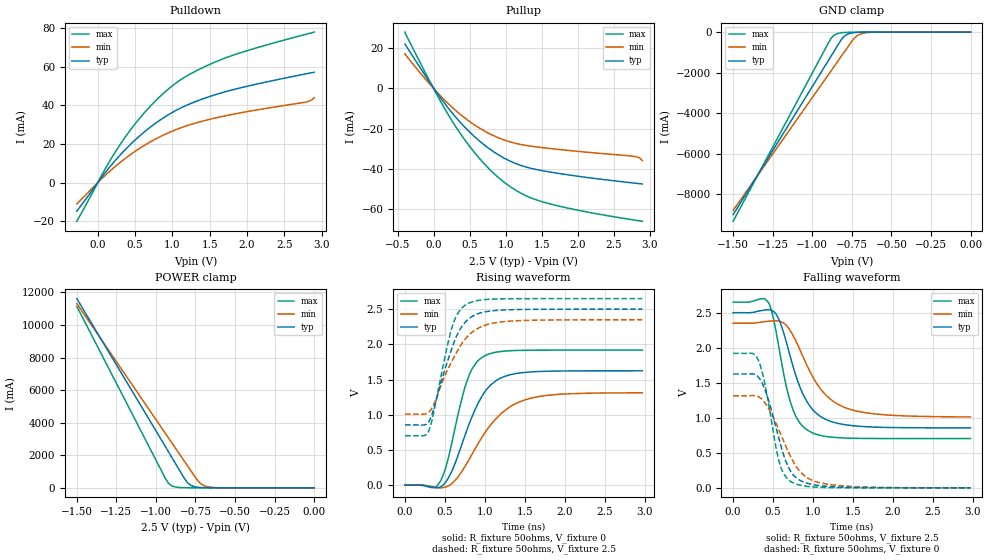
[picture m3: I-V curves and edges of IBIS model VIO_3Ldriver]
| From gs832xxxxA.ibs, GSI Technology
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|  signals   DQA1-DQA9, DQB1-DQB9, DQC1-DQC9, DQD1-DQD9
[Model]   VIO_3Ldriver
Model_type   I/O
Polarity   Non-Inverting
Vinl  =   0.80v
Vinh  =   2.00v
Vmeas =   1.25v
Cref  =   0pF
Rref  =   50
Vref  =   1.25v
|  variable   typ   min   max
C_comp   3.0pF   2.5pF   3.5pF
|  variable   typ   min   max
[Temperature Range]   50   0   100
|  variable   typ   min   max
[Voltage Range]   2.5   2.35   2.65
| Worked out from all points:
|   slope of the pulldown table from 0 to 0.375 V, typ, clamps not added: 21.6 ohm
|   slope of the pullup table from 0 to 0.375 V, typ, clamps not added: 21.9 ohm
|   GND clamp passes 1 mA (typ) near -0.58 V on its own axis
|   POWER clamp passes 1 mA (typ) near -0.61 V on its own axis
|   rising waveform, R_fixture 50ohms, V_fixture 0: 20-80 % time 352ps typ, 488ps min, 252ps max; typ from 0 V to 1.62 V
|   rising waveform, R_fixture 50ohms, V_fixture 2.5: 20-80 % time 284ps typ, 353ps min, 224ps max; typ from 0.855 V to 2.5 V
|   falling waveform, R_fixture 50ohms, V_fixture 2.5: 20-80 % time 308ps typ, 411ps min, 225ps max; typ from 2.5 V to 0.856 V
|   falling waveform, R_fixture 50ohms, V_fixture 0: 20-80 % time 250ps typ, 334ps min, 186ps max; typ from 1.62 V to 0 V
[Pulldown]
| voltage   typ   min   max
-280mV    -14.72mA   -10.94mA   -19.96mA
105mV     5.397mA    3.94mA     7.47mA
350mV     16.36mA    11.99mA    22.57mA
525mV     22.94mA    16.83mA    31.61mA
665mV     27.53mA    20.21mA    37.92mA
980mV     35.91mA    26.36mA    49.51mA
1.295V    41.73mA    30.66mA    57.37mA
1.715V    47.1mA     34.66mA    64.61mA
2.1V      50.75mA    37.42mA    69.45mA
2.8V      56.38mA    41.82mA    76.89mA
2.87V     56.91mA    42.86mA    77.59mA
2.9V      57.14mA    44.01mA    77.94mA
[Pullup]
| voltage (VDDQ-Vout) typ   min   max
-400mV    21.9mA     17.14mA    27.88mA
25mV      -1.299mA   -1.191mA   -2.024mA
305mV     -14.32mA   -11.03mA   -19.02mA
480mV     -21.05mA   -16.03mA   -27.95mA
655mV     -26.75mA   -20.17mA   -35.62mA
970mV     -34.47mA   -25.52mA   -46.36mA
1.25V     -38.71mA   -28.14mA   -52.74mA
1.53V     -40.98mA   -29.49mA   -56.47mA
2.02V     -43.68mA   -31.32mA   -60.56mA
2.755V    -46.86mA   -33.62mA   -65.13mA
2.825V    -47.14mA   -34.08mA   -65.52mA
2.895V    -47.42mA   -35.78mA   -65.9mA
[GND Clamp]
| voltage   typ   min   max
-1.5V     -9.007A    -8.796A    -9.334A
-900mV    -1.426A    -2.122A    -562.9mA
-880mV    -1.174A    -1.9A      -292.9mA
-860mV    -921.1mA   -1.678A    -142.5mA
-820mV    -416.2mA   -1.233A    -38.58mA
-800mV    -222mA     -1.011A    -23.51mA
-780mV    -116.3mA   -788.8mA   -16.2mA
-740mV    -33.04mA   -348.7mA   -9.876mA
-720mV    -18.57mA   -198.2mA   -8.142mA
-680mV    -6.87mA    -61.92mA   -5.539mA
-580mV    -1.002mA   -3.885mA   -1.438mA
0V        -532.9pA   -960.9pA   -479.8pA
[POWER Clamp]
| voltage (VDDQ-Vout) typ   min   max
-1.5V     11.62A     11.31A     11.14A
-940mV    2.526A     3.337A     574.2mA
-920mV    2.201A     3.052A     270.7mA
-900mV    1.877A     2.767A     123.3mA
-880mV    1.552A     2.482A     56.51mA
-820mV    578.6mA    1.628A     8.04mA
-800mV    303.9mA    1.344A     5.265mA
-760mV    77.74mA    774.1mA    2.987mA
-720mV    20.11mA    274.2mA    1.963mA
-680mV    5.757mA    82.61mA    1.268mA
-580mV    536.8uA    4.105mA    264.2uA
0V        760.6pA    2.222nA    464.4pA
[Ramp]
| voltage   typ   min   max
dV/dt_r   1.41/142p   1.22/179p   1.66/116p
dV/dt_f   1.36/139p   1.15/172p   1.63/115p
R_load  =   50ohms
[Rising Waveform]
C_fixture =   0.0pf
R_fixture =   50ohms
V_fixture =   0
| Time   V(typ)   V(min)   V(max)
0s        7.245nV    16.29nV    5.043nV
360ps     -34.32mV   -25.8mV    -32.85mV
450ps     -21.93mV   -37.96mV   68.51mV
570ps     160.3mV    8.732mV    519.7mV
780ps     800.4mV    321.9mV    1.494V
900ps     1.128V     561.4mV    1.753V
990ps     1.312V     727.3mV    1.833V
1.26ns    1.55V      1.07V      1.905V
1.56ns    1.607V     1.231V     1.917V
2.97ns    1.625V     1.312V     1.919V
[Rising Waveform]
C_fixture =   0.0pf
R_fixture =   50ohms
V_fixture =   2.5
V_fixture_min =   2.35
V_fixture_max =   2.65
| Time   V(typ)   V(min)   V(max)
0s        855.1mV    1.009V     703mV
240ps     854.5mV    1.008V     703.2mV
300ps     902mV      1.035V     774.3mV
540ps     1.786V     1.655V     2.029V
600ps     1.987V     1.79V      2.286V
690ps     2.217V     1.974V     2.489V
780ps     2.346V     2.109V     2.576V
960ps     2.451V     2.253V     2.631V
1.23ns    2.488V     2.322V     2.647V
2.97ns    2.5V       2.35V      2.65V
[Falling Waveform]
C_fixture =   0.0pf
R_fixture =   50ohms
V_fixture =   2.5
V_fixture_min =   2.35
V_fixture_max =   2.65
| Time   V(typ)   V(min)   V(max)
0s        2.5V       2.35V      2.65V
390ps     2.537V     2.371V     2.701V
450ps     2.543V     2.379V     2.631V
570ps     2.41V      2.38V      2.02V
720ps     1.851V     2.235V     1.211V
840ps     1.426V     1.959V     918.7mV
960ps     1.167V     1.661V     803.9mV
1.2ns     957.2mV    1.281V     727.5mV
1.5ns     886.7mV    1.109V     707.7mV
2.97ns    855.5mV    1.012V     703.2mV
[Falling Waveform]
C_fixture =   0.0pf
R_fixture =   50ohms
V_fixture =   0
| Time   V(typ)   V(min)   V(max)
0s        1.625V     1.313V     1.919V
240ps     1.627V     1.317V     1.918V
300ps     1.599V     1.309V     1.859V
390ps     1.424V     1.225V     1.524V
570ps     716.5mV    832.8mV    398.1mV
630ps     473.1mV    671mV      204.7mV
720ps     234.2mV    442.7mV    90mV
900ps     75.13mV    165.3mV    25.3mV
1.14ns    24.35mV    59.23mV    5.159mV
2.97ns    11.38uV    289uV      -9.878nV
